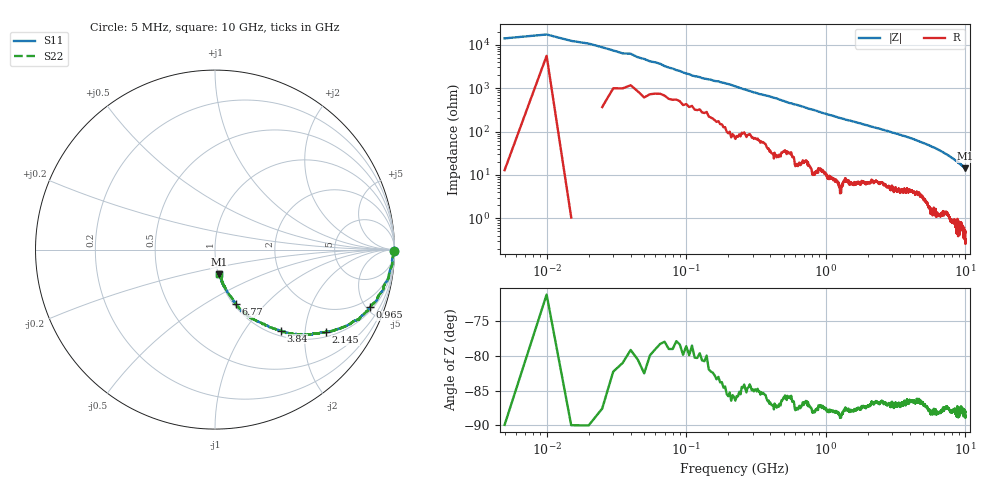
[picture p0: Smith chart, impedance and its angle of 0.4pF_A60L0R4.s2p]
! Amotech Co.,Ltd.
! http://www.amotech.co.kr/
! Part Number: A60L0R4
! These Parameters are Measured in Series Mode Connection
! Operation Temp=25[degC], DC Bias Voltage=0[V]
! Freq. Start=5[MHz] Stop=10[GHz], 2000[Steps]
! Date: Monday, July 14, 2020, 09:25:12
# GHZ S RI R 50.000000
!Freq.(Hz) S11(Real) S11(Imag) S21(Real) S21(Imag) S12(Real) S12(Imag) S22(Real) S22(Imag)
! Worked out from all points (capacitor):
!   2000 points, 5 MHz to 10 GHz, reference 50 ohm
!   read as one part in series: C = 729 fF near 55 MHz
!   lowest |Z| = 14.1 ohm at 9.99 GHz (marker M1)
!   S11 on the Smith chart (normalised r, x): 5 MHz: open; 965 MHz: 1.24, -5.27; 2.145 GHz: 1.15, -2.58; 3.84 GHz: 1.09, -1.49; 6.77 GHz: 1.03, -0.69; 10 GHz: 1.01, -0.28
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0.005  0.9999 -0.00716  5.78e-05 0.00716  5.78e-05 0.00716  0.9999 -0.00716
0.035  0.9973 -0.0155  0.0027 0.0155  0.0027 0.0155  0.9973 -0.0155
0.08  0.9921 -0.0342  0.00789 0.0342  0.00789 0.0342  0.9921 -0.0342
0.115  0.9884 -0.0513  0.0116 0.0513  0.0116 0.0513  0.9884 -0.0513
0.16  0.987 -0.0665  0.013 0.0665  0.013 0.0665  0.987 -0.0665
0.27  0.9793 -0.1068  0.0207 0.1068  0.0207 0.1068  0.9793 -0.1068
0.355  0.9693 -0.1365  0.0307 0.1365  0.0307 0.1365  0.9693 -0.1365
0.555  0.94 -0.2049  0.06 0.2049  0.06 0.2049  0.94 -0.2049
0.75  0.9085 -0.2656  0.0915 0.2656  0.0915 0.2656  0.9085 -0.2656
0.965  0.8634 -0.3211  0.1366 0.3211  0.1366 0.3211  0.8634 -0.3211
1.275  0.8018 -0.3886  0.1982 0.3886  0.1982 0.3886  0.8018 -0.3886
1.675  0.7123 -0.4327  0.2877 0.4327  0.2877 0.4327  0.7123 -0.4327
2.145  0.6181 -0.4582  0.3819 0.4582  0.3819 0.4582  0.6181 -0.4582
3.34  0.4267 -0.4678  0.5733 0.4678  0.5733 0.4678  0.4267 -0.4678
3.84  0.3661 -0.4514  0.6339 0.4514  0.6339 0.4514  0.3661 -0.4514
5.005  0.2387 -0.4006  0.7613 0.4006  0.7613 0.4006  0.2387 -0.4006
5.8  0.1699 -0.3608  0.8301 0.3608  0.8301 0.3608  0.1699 -0.3608
6.67  0.1206 -0.3094  0.8794 0.3094  0.8794 0.3094  0.1206 -0.3094
6.77  0.1157 -0.3018  0.8843 0.3018  0.8843 0.3018  0.1157 -0.3018
8.335  0.0554 -0.2128  0.9446 0.2128  0.9446 0.2128  0.0554 -0.2128
9.99  0.0225 -0.1373  0.9775 0.1373  0.9775 0.1373  0.0225 -0.1373
10  0.0226 -0.1374  0.9774 0.1374  0.9774 0.1374  0.0226 -0.1374
